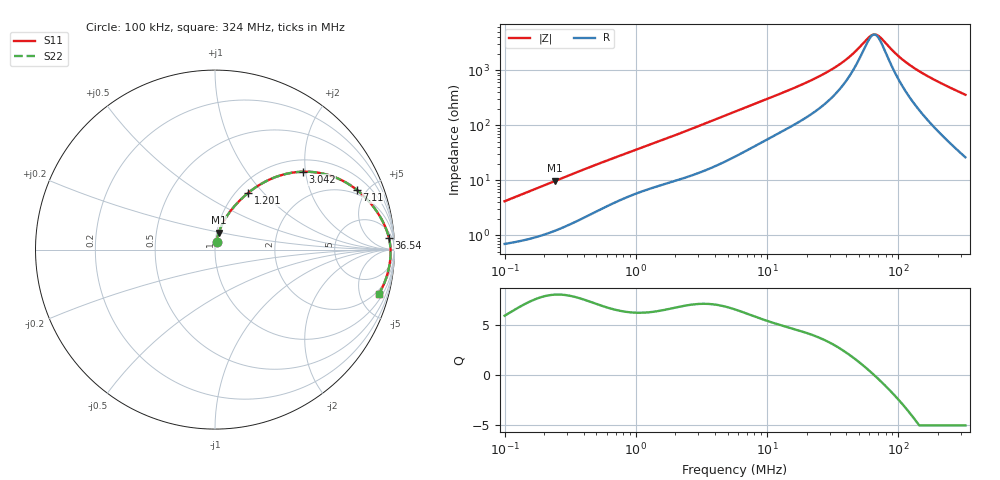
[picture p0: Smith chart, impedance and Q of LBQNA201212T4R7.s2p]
! LBQNA201212T4R7  S-PARAMETER MODEL  ( General Type )
! Model Generated by TAIYO YUDEN Corporation (http://www.ty-top.com)
! Version 1.0
! TAIYO YUDEN Control No. 191025NI43SB-FBB
! Copyright(c) 2019 TAIYO YUDEN CO.,LTD. All Rights Reserved.
! Product Description (link to TY-COMPAS)
! https://ds.yuden.co.jp/TYCOMPAS/or/detail?pn=LBQNA201212T4R7M&u=M
! Products Name : Inductors
! Characteristics :
!  Inductance : 4.7 uH , SRF(min) : 45 MHz , DC Resistance(max) : 0.52 Ohm
!  Rated Current : Saturation :300 mA , Temp Rise : 430 mA (20 degC)
!  Case Size : 2.0 x 1.25 / 0.079 x 0.049 [mm/inch] , Thickness : 1.25 / 0.049 [mm/inch]
!  (Conditions: Temperature = 25 degC , DC Bias Current/Voltage = 0A / 0V)
! External Node Assignments :
!  1  o---GGG---o  2
! GND o---------o GND
! Frequency Range : 0.1MHz  -  324.04089MHz  [ 402 STEP ]
# MHz S RI R 50
! Freq[MHz].  S11 Real  S11 Imag  S21 Real  S21 Imag  S12 Real  S12 Imag  S22 Real  S22 Imag
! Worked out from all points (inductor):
!   401 points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, 100 kHz to 324 MHz, reference 50 ohm
!   read as one part in series: L = 6.45 uH near 104.1 kHz
!   highest Q = 7.97 at 243.3 kHz (marker M1), where L = 6.33 uH
!   self-resonance near 65.32 MHz
!   S11 on the Smith chart (normalised r, x): 100 kHz: 1.01, +0.08; 1.201 MHz: 1.13, +0.83; 3.042 MHz: 1.27, +1.93; 7.11 MHz: 1.71, +4.29; 36.54 MHz: 11, +25; 324 MHz: 1.52, -7.13
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0.1  0.00855 0.0403  0.9915 -0.0403  0.9915 -0.0403  0.00855 0.0403
0.243313  0.0209 0.0935  0.9791 -0.0935  0.9791 -0.0935  0.0209 0.0935
0.38728  0.0404 0.1415  0.9596 -0.1415  0.9596 -0.1415  0.0404 0.1415
0.710102  0.0956 0.2266  0.9044 -0.2266  0.9044 -0.2266  0.0956 0.2266
1.200907  0.1846 0.3156  0.8154 -0.3156  0.8154 -0.3156  0.1846 0.3156
1.499861  0.2386 0.3547  0.7614 -0.3547  0.7614 -0.3547  0.2386 0.3547
3.042485  0.4885 0.4339  0.5115 -0.4339  0.5115 -0.4339  0.4885 0.4339
4.119798  0.6119 0.4208  0.3881 -0.4208  0.3881 -0.4208  0.6119 0.4208
5.692459  0.7269 0.3752  0.2731 -0.3752  0.2731 -0.3752  0.7269 0.3752
7.109538  0.7895 0.3334  0.2105 -0.3334  0.2105 -0.3334  0.7895 0.3334
11.78295  0.8852 0.235  0.1148 -0.235  0.1148 -0.235  0.8852 0.235
22.04577  0.9461 0.1328  0.0539 -0.1328  0.0539 -0.1328  0.9461 0.1328
36.53742  0.9688 0.0663  0.0312 -0.0663  0.0312 -0.0663  0.9688 0.0663
45.63304  0.974 0.0402  0.026 -0.0402  0.026 -0.0402  0.974 0.0402
59.3436  0.9774 0.0107  0.0226 -0.0107  0.0226 -0.0107  0.9774 0.0107
64.33982  0.9779 0.00168  0.0221 -0.00168  0.0221 -0.00168  0.9779 0.00168
71.18072  0.9782 -0.00959  0.0218 0.00959  0.0218 0.00959  0.9782 -0.00959
85.37896  0.978 -0.0303  0.022 0.0303  0.022 0.0303  0.978 -0.0303
106.6332  0.9761 -0.057  0.0239 0.057  0.0239 0.057  0.9761 -0.057
141.5022  0.9705 -0.0949  0.0295 0.0949  0.0295 0.0949  0.9705 -0.0949
207.7384  0.9542 -0.1571  0.0458 0.1571  0.0458 0.1571  0.9542 -0.1571
324.0409  0.9117 -0.2494  0.0883 0.2494  0.0883 0.2494  0.9117 -0.2494
